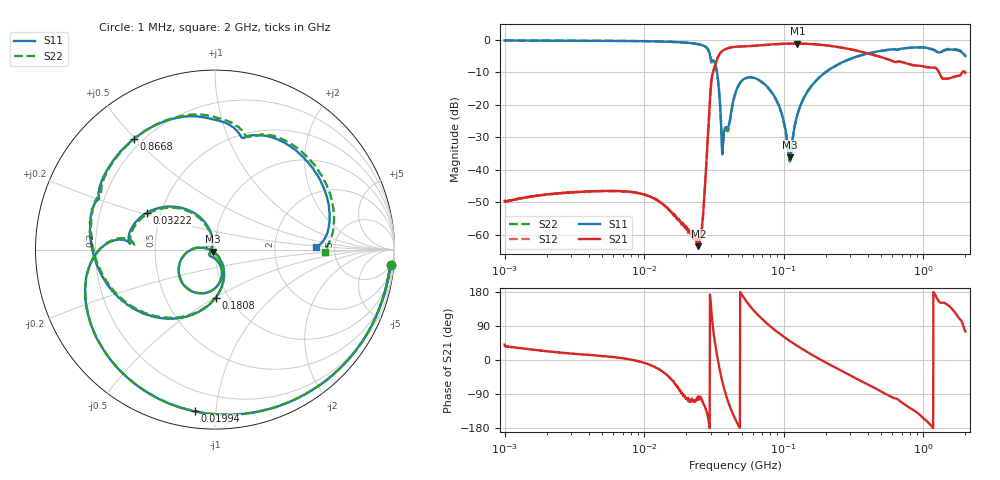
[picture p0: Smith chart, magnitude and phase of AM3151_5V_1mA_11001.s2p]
! Date/Time: Fri Jun 26 11:06:21 2020
! Network Analyzer:  Rev:
! Sweep from 1000000.0 to 2000000000.0, 1601 Points ! Power Supply: 0 V, 0 A
# HZ S DB R 50
!freq MagS11 AngS11 MagS21 AngS21 MagS12 AngS12 MagS22 AngS22
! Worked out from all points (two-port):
!   1601 points, 1 MHz to 2 GHz, reference 50 ohm
!   highest |S21| = -1.10 dB at 125.4 MHz (marker M1); lowest = -63.5 dB at 24.46 MHz (marker M2)
!   |S21| within 3 dB of the highest: 34.98 MHz to 394.2 MHz (359.2 MHz wide, 167 % of centre)
!   lowest |S11| = -36.1 dB at 110.3 MHz (marker M3), VSWR 1.03, Z = 49 - j1.21 ohm
!   |S11| at or under -10 dB: 33.21 MHz to 198.2 MHz (165 MHz wide, 143 % of centre)
!   |S22| runs from -37.4 to -0.2 dB; largest |S21 - S12| = 0.0069
!   S11 on the Smith chart (normalised r, x): 1 MHz: 5, -22; 19.94 MHz: 0.09, -0.88; 32.22 MHz: 0.42, +0.21; 180.8 MHz: 0.87, -0.50; 866.8 MHz: 0.17, +0.50; 2 GHz: 3.57, +0.12
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1000000  -0.16 -4.9  -49.49 40.9  -49.82 36.1  -0.16 -5.0
3555161  -0.23 -16.5  -46.73 15.0  -46.74 14.7  -0.23 -16.5
1.263916e7  -0.45 -58.9  -49.57 -23.5  -49.54 -23.2  -0.46 -59.0
1.994252e7  -0.84 -97.2  -57.68 -99.4  -58.27 -101.5  -0.85 -97.4
2.446217e7  -1.32 -127.0  -63.46 -99.2  -62.14 -109.0  -1.33 -127.4
2.626893e7  -1.67 -142.4  -55.38 -110.6  -54.80 -112.0  -1.70 -142.9
2.986397e7  -5.43 174.0  -15.79 156.8  -15.78 156.8  -5.84 172.9
3.222237e7  -7.27 151.8  -7.78 43.3  -7.78 43.2  -7.31 153.3
3.443828e7  -16.11 109.6  -4.55 -18.0  -4.55 -17.9  -15.97 111.8
3.680657e7  -31.29 -147.4  -3.21 -66.5  -3.21 -66.5  -31.13 -159.3
4.493426e7  -16.38 -75.9  -2.10 -156.1  -2.10 -156.1  -16.51 -74.6
5.779954e7  -11.48 -124.3  -1.87 140.7  -1.87 140.6  -11.55 -124.2
7.649789e7  -14.50 -166.0  -1.48 95.0  -1.48 95.1  -14.59 -166.6
1.102838e8  -36.07 -128.5  -1.14 50.4  -1.13 50.4  -37.41 -124.0
1.253766e8  -22.93 -62.5  -1.10 36.9  -1.12 36.9  -22.88 -60.7
1.589914e8  -13.97 -78.1  -1.28 14.0  -1.27 13.9  -14.01 -77.9
1.807501e8  -11.42 -89.3  -1.46 2.3  -1.47 2.3  -11.44 -89.5
3.181212e8  -5.40 -138.6  -3.07 -45.7  -3.09 -46.0  -5.47 -139.7
5.652395e8  -3.01 169.7  -6.08 -93.9  -6.04 -94.0  -3.02 167.7
8.667936e8  -2.33 126.1  -7.89 -134.2  -7.84 -134.3  -2.32 123.7
1.461712e9  -3.07 62.4  -11.93 147.4  -11.81 147.3  -2.88 60.4
2e9  -4.99 1.2  -10.15 75.2  -10.30 74.7  -4.29 -1.5
